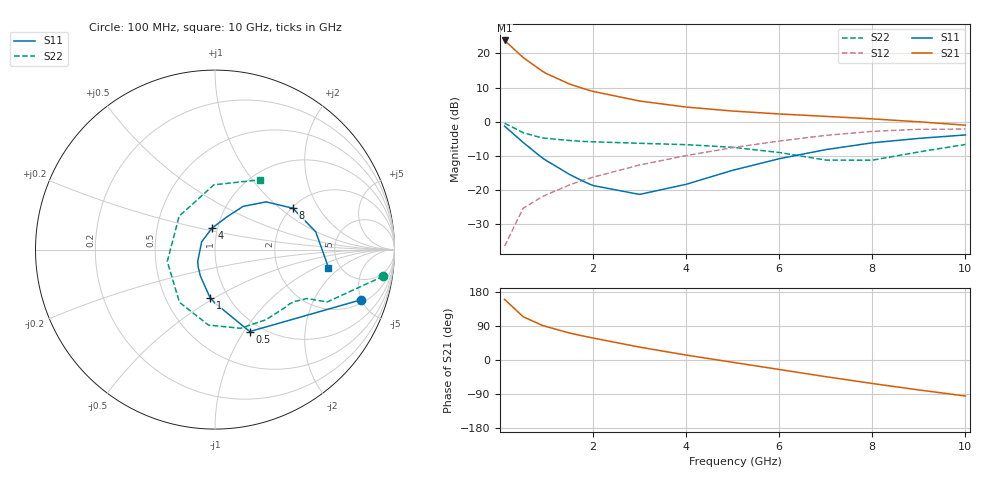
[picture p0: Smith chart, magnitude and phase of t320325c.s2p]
!AT-32032
!S-PARAMETERS at Vce=5V  Ic=5mA.  LAST UPDATED 05-29-98
# ghz s ma r 50
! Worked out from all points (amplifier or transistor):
!   15 points, 100 MHz to 10 GHz, reference 50 ohm
!   highest |S21| = 23.8 dB at 100 MHz (marker M1)
!   |S21| within 3 dB of that: start of sweep to 338.8 MHz
!   unconditionally stable (mu >= 1): 1.392 GHz to 3.137 GHz
!   at 900 MHz: K = 0.90, MSG = 18.5 dB, |S12| = -22.0 dB
!   at 3 GHz: K = 1.01, MAG = 8.8 dB, |S12| = -12.7 dB
!   at 10 GHz: K = 0.92, MSG = 0.6 dB, |S12| = -2.1 dB
!   lowest NFmin = 1.00 dB at 900 MHz
!   S11 on the Smith chart (normalised r, x): 100 MHz: 2.30, -4.94; 500 MHz: 0.88, -1.06; 1 GHz: 0.82, -0.47; 4 GHz: 0.94, +0.23; 8 GHz: 2.03, +1.23; 10 GHz: 4.06, -1.38
0.1  0.86 -19.0  15.52 160.0  0.015 80.0  0.949 -9.0
0.5  0.496 -67.0  8.705 114.0  0.054 63.0  0.69 -25.0
0.9  0.298 -90.0  5.569 92.0  0.079 61.0  0.58 -28.0
1  0.269 -96.0  5.067 88.0  0.085 61.0  0.57 -29.0
1.5  0.168 -119.0  3.558 71.0  0.119 59.0  0.53 -33.0
1.8  0.133 -135.0  3.046 63.0  0.14 58.0  0.514 -36.0
2  0.116 -146.0  2.782 58.0  0.154 57.0  0.508 -39.0
3  0.086 150.0  2.011 34.0  0.232 48.0  0.483 -54.0
4  0.121 98.0  1.64 13.0  0.319 37.0  0.461 -72.0
5  0.194 70.0  1.434 -6.0  0.417 23.0  0.422 -95.0
6  0.287 57.0  1.3 -25.0  0.521 8.0  0.354 -124.0
7  0.39 43.0  1.198 -44.0  0.631 -10.0  0.274 -166.0
8  0.491 28.0  1.101 -62.0  0.722 -30.0  0.273 137.0
9  0.57 10.0  0.997 -79.0  0.774 -51.0  0.361 91.0
10  0.64 -9.0  0.891 -95.0  0.781 -72.0  0.464 57.0
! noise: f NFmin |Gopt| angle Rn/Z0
0.9  1  0.38  52  0.23
1.8  1.2  0.335  124  0.13
2  1.3  0.33  140  0.11
2.5  1.4  0.35  179  0.09
3  1.6  0.4  -146  0.12
3.5  1.8  0.47  -118  0.23
4  2  0.54  -92  0.44
